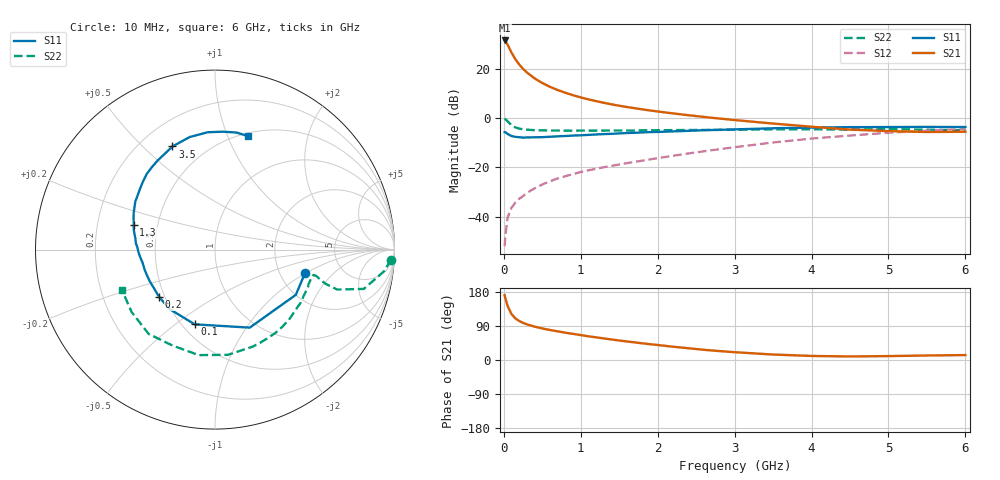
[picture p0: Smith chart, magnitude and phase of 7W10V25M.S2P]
! Infineon Technologies  Discrete & RF Semiconductors
! BFS17W
! Si NPN RF Bipolar Junction Transistor in SOT323
! VCE = 10 V  IC = 25 mA
! Common Emitter S-Parameters:  August  1999
# GHz  S  MA  R  50
!  f  S11  S21  S12  S22
! GHz  MAG  ANG  MAG  ANG  MAG  ANG  MAG  ANG
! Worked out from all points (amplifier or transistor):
!   36 points, 10 MHz to 6 GHz, reference 50 ohm
!   highest |S21| = 31.6 dB at 10 MHz (marker M1)
!   |S21| within 3 dB of that: start of sweep to 69.04 MHz
!   unconditionally stable (mu >= 1): 295.2 MHz to 1.954 GHz; 5.706 GHz to end of sweep
!   at 250 MHz: K = 0.98, MSG = 25.9 dB, |S12| = -31.7 dB
!   at 1.4 GHz: K = 1.13, MAG = 10.3 dB, |S12| = -19.4 dB
!   at 6 GHz: K = 1.02, MAG = -1.5 dB, |S12| = -4.4 dB
!   S11 on the Smith chart (normalised r, x): 10 MHz: 2.75, -0.98; 100 MHz: 0.58, -0.59; 200 MHz: 0.47, -0.30; 1.3 GHz: 0.36, +0.13; 3.5 GHz: 0.33, +0.62; 6 GHz: 0.53, +1.19
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0.01  0.5182 -14.6  37.83 171.2  0.0025 80.7  0.9821 -3.3
0.02  0.5162 -29.2  36.86 162.7  0.0041 77.0  0.9497 -7.3
0.05  0.4759 -66.0  30.77 141.9  0.0097 71.2  0.8575 -14.8
0.1  0.4315 -105.2  21.37 121.2  0.0151 60.8  0.7165 -18.1
0.15  0.4165 -127.0  15.72 109.8  0.0193 60.1  0.646 -17.2
0.2  0.4084 -139.5  12.29 102.9  0.023 64.5  0.6117 -16.0
0.25  0.4023 -148.1  10.02 97.9  0.026 64.1  0.5916 -15.0
0.3  0.4045 -154.6  8.445 94.1  0.0304 66.5  0.582 -14.6
0.4  0.4076 -163.7  6.421 88.0  0.0374 68.7  0.568 -14.4
0.5  0.41 -169.6  5.17 83.3  0.0449 69.4  0.5637 -14.9
0.6  0.4183 -174.0  4.314 79.2  0.0521 70.6  0.5601 -15.9
0.7  0.4264 -177.9  3.724 75.6  0.0594 71.5  0.5587 -17.1
0.9  0.4425 175.4  2.915 68.9  0.0729 72.5  0.5557 -20.3
1.1  0.4563 169.1  2.405 62.5  0.0869 73.1  0.5574 -24.0
1.3  0.4735 163.1  2.049 56.9  0.1007 73.8  0.5576 -28.1
1.6  0.498 155.4  1.679 48.9  0.1215 74.9  0.5602 -34.4
2.2  0.537 141.3  1.246 35.0  0.1718 76.4  0.5704 -48.6
2.8  0.5784 127.5  0.98 23.6  0.2331 74.8  0.5767 -64.1
3.5  0.6217 112.4  0.775 14.4  0.3198 69.9  0.5905 -83.0
4.5  0.6551 93.6  0.584 9.3  0.4418 57.7  0.5846 -113.8
5.5  0.6631 79.5  0.522 11.9  0.5546 44.5  0.5803 -143.2
6  0.6584 73.8  0.529 13.0  0.6002 37.7  0.5652 -156.6
